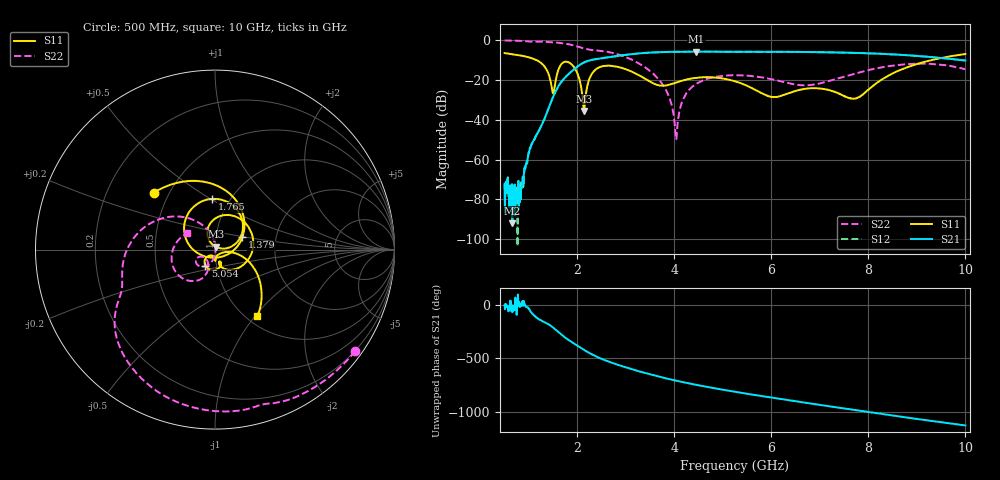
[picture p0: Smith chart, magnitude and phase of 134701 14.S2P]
!  2-Port S-parameters saved by WinCal
! VAR MeasName=S-Parameters (CALIBRATED_DATA) read from VNA (N5242A)
! VAR MeasDate=2013-7-3 16:29:34
! VAR NAME=134701 14
! VAR FILENAME=134701 14.S2P
! VAR DATE=2013-7-3 16:29:34
! VAR PHYS_PORTS=1,2
# Hz S MA R 50
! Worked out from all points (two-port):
!   1601 points, 500 MHz to 10 GHz, reference 50 ohm
!   highest |S21| = -5.94 dB at 4.454 GHz (marker M1); lowest = -92.0 dB at 660.3 MHz (marker M2)
!   |S21| within 3 dB of the highest: 2.588 GHz to 9.423 GHz (6.835 GHz wide, 114 % of centre)
!   lowest |S11| = -35.7 dB at 2.139 GHz (marker M3), VSWR 1.03, Z = 50.4 + j1.59 ohm
!   |S11| at or under -10 dB: 1.142 GHz to 9.334 GHz (8.192 GHz wide, 156 % of centre)
!   |S22| runs from -49.9 to -0.3 dB; largest |S21 - S12| = 0.0028
!   S11 on the Smith chart (normalised r, x): 500 MHz: 0.41, +0.34; 1.379 GHz: 1.34, +0.19; 1.765 GHz: 0.83, +0.51; 5.054 GHz: 0.88, -0.16; 10 GHz: 1.12, -1.03
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5e8  0.4653 136.9  0.0002466 -1.2  0.0002449 -15.8  0.963 -35.9
6.603125e8  0.4373 123.9  2.514e-05 -70.7  0.0001567 -11.1  0.9535 -47.2
8.384375e8  0.403 108.0  0.0001987 -13.5  0.0002827 9.3  0.9381 -60.0
1.040312e9  0.3522 86.5  0.002133 -67.9  0.002171 -67.8  0.9021 -73.4
1.37875e9  0.1666 24.3  0.0154 -176.0  0.01538 -175.8  0.8882 -97.6
1.503438e9  0.04538 -92.7  0.03797 145.9  0.03795 145.6  0.8675 -107.2
1.764688e9  0.2831 93.0  0.1194 49.0  0.1192 49.1  0.7943 -127.5
2.085312e9  0.05705 6.1  0.2505 -45.7  0.25 -45.7  0.6319 -150.0
2.13875e9  0.01638 73.6  0.2709 -60.7  0.2703 -60.7  0.6054 -152.5
2.287188e9  0.1325 105.9  0.3119 -98.8  0.3109 -98.9  0.558 -158.1
2.524688e9  0.2188 55.3  0.3482 -148.0  0.3476 -148.0  0.5204 -170.9
3.670625e9  0.07292 -72.3  0.4897 52.6  0.4895 52.7  0.104 108.2
4.03875e9  0.085 -66.3  0.5019 13.8  0.502 13.7  0.00321 -13.6
4.193125e9  0.09706 -71.7  0.5036 -1.1  0.5036 -1.2  0.03494 -93.4
4.454375e9  0.1117 -86.1  0.5047 -25.0  0.5048 -25.1  0.07902 -108.8
5.054062e9  0.1043 -121.1  0.5015 -74.4  0.5017 -74.4  0.1268 -134.2
5.25e9  0.09096 -129.8  0.5008 -89.3  0.5009 -89.4  0.1296 -140.7
6.015938e9  0.03696 -114.0  0.5002 -144.2  0.4997 -144.2  0.1024 -155.9
6.835312e9  0.06127 -88.3  0.4937 159.8  0.4939 159.8  0.07447 -127.1
7.72e9  0.0337 -51.7  0.4712 101.4  0.4709 101.4  0.1412 -109.8
8.420625e9  0.1281 -11.1  0.436 55.6  0.435 55.6  0.2182 -126.7
1e10  0.4398 -57.4  0.3028 -42.1  0.3038 -41.8  0.1823 150.4
